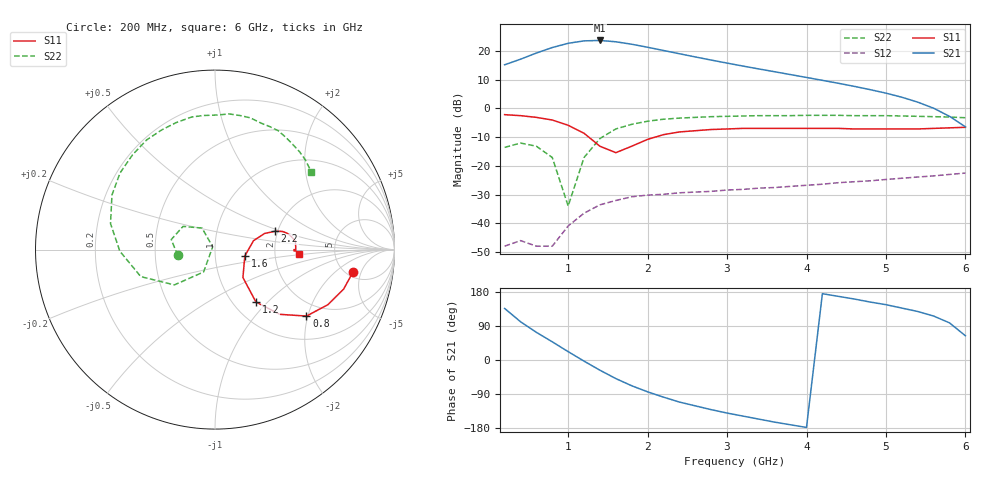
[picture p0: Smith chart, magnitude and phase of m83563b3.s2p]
!	MGA-83563 S PARAMETERS
!	Vd = 3 V L=8.2 nH  LAST UPDATED 10-15-97
# ghz	s ma r	50
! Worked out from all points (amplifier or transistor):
!   30 points, 200 MHz to 6 GHz, reference 50 ohm
!   highest |S21| = 23.7 dB at 1.4 GHz (marker M1)
!   |S21| within 3 dB of that: 744.1 MHz to 2.112 GHz (1.368 GHz wide, 95.8 % of centre)
!   unconditionally stable (mu >= 1): start of sweep to end of sweep
!   at 1.2 GHz: K = 1.99, MAG = 24.3 dB, |S12| = -36.5 dB
!   at 3.2 GHz: K = 1.23, MAG = 18.6 dB, |S12| = -28.2 dB
!   at 6 GHz: K = 5.45, MAG = -2.3 dB, |S12| = -22.5 dB
!   S11 on the Smith chart (normalised r, x): 200 MHz: 5.79, -3.61; 800 MHz: 1.60, -1.96; 1.2 GHz: 1.27, -0.86; 1.6 GHz: 1.39, -0.10; 2.2 GHz: 1.94, +0.45; 6 GHz: 2.76, -0.17
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0.2  0.78 -9.0  5.77 136.0  0.004 56.0  0.21 -171.0
0.4  0.75 -17.0  7.21 101.0  0.005 41.0  0.25 167.0
0.6  0.7 -26.0  9.24 73.0  0.004 50.0  0.22 144.0
0.8  0.63 -36.0  11.52 48.0  0.004 95.0  0.14 121.0
1  0.51 -45.0  13.65 22.0  0.009 111.0  0.02 130.0
1.2  0.37 -52.0  15.05 -3.0  0.015 105.0  0.14 -117.0
1.4  0.22 -45.0  15.3 -27.0  0.021 94.0  0.3 -139.0
1.6  0.17 -12.0  14.51 -49.0  0.025 83.0  0.44 -160.0
1.8  0.22 13.0  13.15 -68.0  0.029 74.0  0.53 -179.0
2  0.29 18.0  11.65 -84.0  0.031 67.0  0.6 166.0
2.2  0.35 17.0  10.23 -98.0  0.032 61.0  0.65 152.0
2.4  0.39 15.0  8.98 -111.0  0.034 57.0  0.68 141.0
2.6  0.41 13.0  7.9 -121.0  0.035 54.0  0.7 131.0
2.8  0.43 10.0  6.97 -131.0  0.036 51.0  0.72 122.0
3  0.44 8.0  6.17 -140.0  0.038 49.0  0.73 114.0
3.2  0.45 6.0  5.48 -148.0  0.039 47.0  0.74 107.0
3.6  0.45 3.0  4.36 -164.0  0.042 43.0  0.75 95.0
4.2  0.45 1.0  3.09 175.0  0.048 38.0  0.76 79.0
4.8  0.44 -1.0  2.13 153.0  0.055 32.0  0.75 66.0
5.2  0.44 -1.0  1.57 137.0  0.061 27.0  0.74 58.0
5.6  0.45 -1.0  1.01 116.0  0.067 22.0  0.72 49.0
6  0.47 -3.0  0.48 64.0  0.075 14.0  0.69 39.0
